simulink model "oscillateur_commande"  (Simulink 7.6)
settings: Solver=ode14x  StartTime=0.0  StopTime=0.02
StopFcn:
  | close all, clc
  | load signaux.mat
  | plot(x(1,:),x(2,:))
  | axis([0 0.016 -.5 5.5])
  | grid
  | title('Oscillateur commandé')
  | xlabel('temps')
libraries: fl_lib x6, elec_lib x3, nesl_utility x3

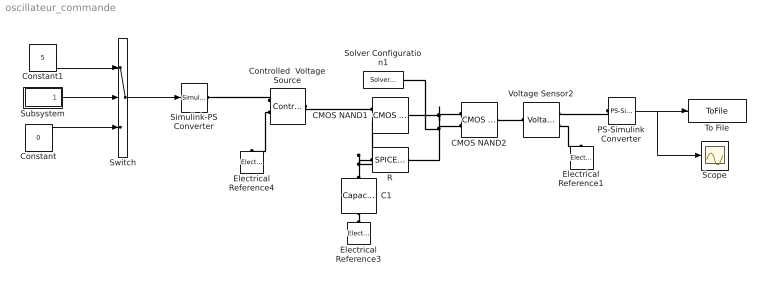
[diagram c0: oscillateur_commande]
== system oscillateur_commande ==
  C1 : fl_lib/Electrical/Electrical Elements/Capacitor  DialogController=NetworkEngine.DynNeDlgSource  SystemSampleTime=-1  c=0.1 nF  v0=0 V  r=1e-6 Ohm  g=0 1/Ohm  i_Log=off  v_Log=off  vc_Log=off  LocalVarNames=|current|voltage|power  LocalVarDescs=|Capacitor current (A)|Voltage across capacitor (V)|Power (W)  LocalVarLogging=[0 0 0]
  CMOS NAND1 : elec_lib/Integrated Circuits/Logic/CMOS NAND  DialogController=NetworkEngine.DynNeDlgSource  SystemSampleTime=-1  V_IL=2 V  V_IH=3 V  C_IN=5 pF  output_type=1  V_OL=0 V  V_OH=5 V  V_CC=5 V  V_meas=5 V  R_OUT=450 Ohm  R_OH=[ 25 250 ] Ohm  I_OH=63 mA  R_OL=[ 30 800 ] Ohm  I_OL=-45 mA  Delay=1.2e-07 s  Ron=5 Ohm  Vf=0.6 V  output_state=1  LocalVarLogging=[]
  CMOS NAND2 : elec_lib/Integrated Circuits/Logic/CMOS NAND  DialogController=NetworkEngine.DynNeDlgSource  SystemSampleTime=-1  V_IL=2 V  V_IH=3 V  C_IN=5 pF  output_type=1  V_OL=0 V  V_OH=5 V  V_CC=5 V  V_meas=5 V  R_OUT=450 Ohm  R_OH=[ 25 250 ] Ohm  I_OH=63 mA  R_OL=[ 30 800 ] Ohm  I_OL=-45 mA  Delay=1.2e-07 s  Ron=5 Ohm  Vf=0.6 V  output_state=1  LocalVarLogging=[]
  Constant : Constant  Value=0
  Constant1 : Constant  Value=5
  Controlled  Voltage Source : fl_lib/Electrical/Electrical Sources/Controlled Voltage Source  DialogController=NetworkEngine.DynNeDlgSource  SystemSampleTime=-1  i_Log=off  v_Log=off  LocalVarNames=|i|v  LocalVarDescs=|i|v  LocalVarLogging=[0 0]
  Electrical Reference1 : fl_lib/Electrical/Electrical Elements/Electrical Reference  DialogController=NetworkEngine.DynNeDlgSource  SystemSampleTime=-1  i_Log=off  LocalVarNames=|i  LocalVarDescs=|i  LocalVarLogging=[]
  Electrical Reference3 : fl_lib/Electrical/Electrical Elements/Electrical Reference  DialogController=NetworkEngine.DynNeDlgSource  SystemSampleTime=-1  i_Log=off  LocalVarNames=|i  LocalVarDescs=|i  LocalVarLogging=[]
  Electrical Reference4 : fl_lib/Electrical/Electrical Elements/Electrical Reference  DialogController=NetworkEngine.DynNeDlgSource  SystemSampleTime=-1  i_Log=off  LocalVarNames=|i  LocalVarDescs=|i  LocalVarLogging=[]
  PS-Simulink Converter : nesl_utility/PS-Simulink Converter  DialogController=NetworkEngine.DynNeUtilDlgSource  SystemSampleTime=-1  PhysicalDomain=network_engine_domain  LeftPortType=input  RightPortType=output  SubClassName=ps_output  Unit=1  AffineConversion=off
  R : elec_lib/Additional Components/SPICE-Compatible Components/Passive Devices/SPICE Resistor  DialogController=NetworkEngine.DynNeDlgSource  SystemSampleTime=-1  SCALE=1  R_param=1  R=220 kOhm  RSH=0 Ohm  LENGTH=1e-06 m  WIDTH=1e-06 m  NARROW=0 m  T_param=1  TC1=0 1/K  TC2=0 1/K^2  TOFFSET=0 K  TFIXED=300.15 K  TMEAS=300.15 K  LocalVarLogging=[]
  Scope : Scope
  Simulink-PS Converter : nesl_utility/Simulink-PS Converter  DialogController=NetworkEngine.DynNeUtilDlgSource  SystemSampleTime=-1  PhysicalDomain=network_engine_domain  LeftPortType=input  RightPortType=output  SubClassName=ps_input  Unit=1  AffineConversion=off  InputFilterTimeConstant=.001  UdotUserProvided=0
  Solver Configuration1 : nesl_utility/Solver Configuration  DialogController=NetworkEngine.DynNeUtilDlgSource  SystemSampleTime=-1  PhysicalDomain=network_engine_domain  LeftPortType=input  RightPortType=generic  SubClassName=solver  Accelerate=off  Profile=off  ResidualTolerance=1e-9  MaxNonlinIter=12  MaxModeIter=2  DoFixedCost=off  UseLocalSampling=off  DoDC=off  LinearAlgebra=Sparse  LocalSolverSampleTime=.001  LocalSolverChoice=NE_BACKWARD_EULER_ADVANCER  UseLocalSolver=off
  Subsystem : Subsystem
  Switch : Switch  Threshold=0.5
  To File : ToFile  Filename=signaux  MatrixName=x
  Voltage Sensor2 : fl_lib/Electrical/Electrical Sensors/Voltage Sensor  DialogController=NetworkEngine.DynNeDlgSource  SystemSampleTime=-1  i1_Log=off  v1_Log=off  LocalVarNames=|i1|v1  LocalVarDescs=|i1|v1  LocalVarLogging=[]
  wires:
  PS-Simulink Converter/1 -> To File/1, Scope/1
  Switch/1 -> Simulink-PS Converter/1
  Constant/1 -> Switch/3
  Subsystem/1(t>0.008) -> Switch/2
  Constant1/1 -> Switch/1
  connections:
  PS-Simulink Converter/LConn1 -- Voltage Sensor2/RConn1
  C1/LConn1 -- Electrical Reference3/LConn1
  Controlled  Voltage Source/LConn1 -- CMOS NAND1/LConn1
  Voltage Sensor2/RConn2 -- Electrical Reference1/LConn1
  CMOS NAND1/RConn1 -- Solver Configuration1/RConn1 -- CMOS NAND2/LConn1 -- R/RConn1 -- CMOS NAND2/LConn2
  C1/RConn1 -- CMOS NAND1/LConn2 -- R/LConn1
  Controlled  Voltage Source/RConn1 -- Simulink-PS Converter/RConn1
  CMOS NAND2/RConn1 -- Voltage Sensor2/LConn1
  Controlled  Voltage Source/RConn2 -- Electrical Reference4/LConn1

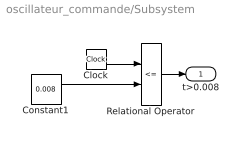
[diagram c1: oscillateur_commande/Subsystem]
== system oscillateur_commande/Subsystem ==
  Clock : Clock
  Constant1 : Constant  Value=0.008
  Relational Operator : RelationalOperator  Operator=<=  OutDataTypeStr=boolean
  t>0.008 : Outport
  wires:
  Clock/1 -> Relational Operator/1
  Constant1/1 -> Relational Operator/2
  Relational Operator/1 -> t>0.008/1
